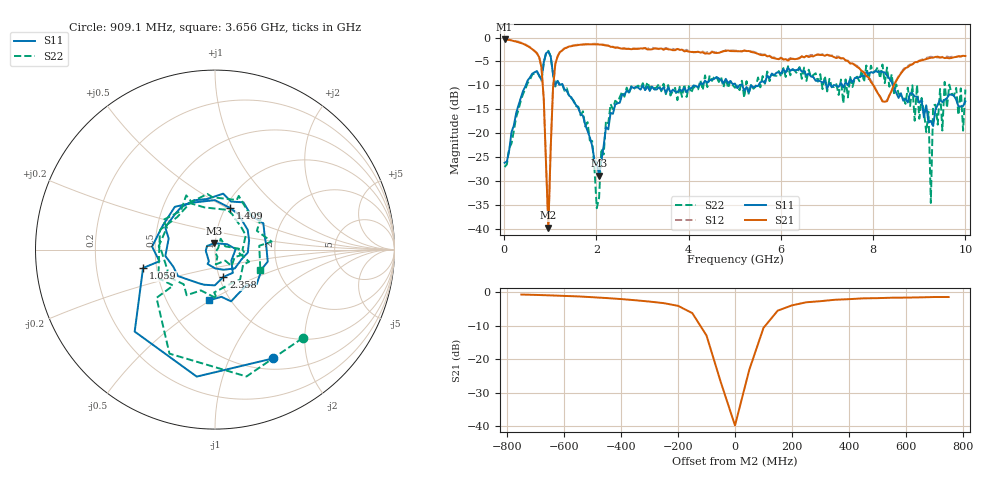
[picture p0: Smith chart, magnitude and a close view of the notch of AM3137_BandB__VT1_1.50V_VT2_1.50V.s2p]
! Date/Time: Tue, Nov 13, 2018 4:51 PM
! Network Analyzer: Agilent Technologies E8364B Rev: A.07.50.67
! Sweep from 0.010 to 10.000 GHz, 201 Points, Sweep Type: LIN
! Power Supply: 1.501 V, 0.000 A
# Hz S DB R 50
!freq MagS11 AngS11 MagS21 AngS21 MagS12 AngS12 MagS22 AngS22
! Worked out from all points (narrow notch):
!   201 points, 10 MHz to 10 GHz, reference 50 ohm
!   highest |S21| = -0.35 dB at 10 MHz (marker M1); lowest = -39.8 dB at 959 MHz (marker M2)
!   notch at M2: 36.4 dB deep, 125 MHz wide at half that depth
!   lowest |S11| = -28.9 dB at 2.058 GHz (marker M3), VSWR 1.07, Z = 49.5 + j3.52 ohm
!   |S11| at or under -10 dB: start of sweep to 468.6 MHz; 1.272 GHz to 4.23 GHz (2.958 GHz wide, 108 % of centre); 8.429 GHz to end of sweep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
!   |S22| runs from -35.7 to -2.8 dB; largest |S21 - S12| = 0.034
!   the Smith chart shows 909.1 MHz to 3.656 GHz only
!   S11 on the Smith chart (normalised r, x): 909.1 MHz: 0.64, -1.47; 1.059 GHz: 0.42, -0.10; 1.409 GHz: 1.05, +0.52; 2.358 GHz: 1.05, -0.33; 3.656 GHz: 0.80, -0.49
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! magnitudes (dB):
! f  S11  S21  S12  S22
! 10 MHz  -26.2  -0.4  -0.3  -27.1
! 759.2 MHz  -7.9  -4.1  -4.0  -8.0
! 909.1 MHz  -3.3  -26.8  -26.6  -3.2
! 959 MHz  -2.9  -39.8  -39.8  -2.8
! 1.059 GHz  -7.7  -10.7  -10.6  -7.5
! 1.409 GHz  -12.2  -1.9  -1.8  -12.3
! 1.708 GHz  -16.3  -1.5  -1.4  -15.4
! 2.058 GHz  -28.9  -1.4  -1.3  -33.6
! 2.108 GHz  -25.8  -1.5  -1.4  -23.2
! 2.358 GHz  -16.0  -2.0  -1.9  -15.0
! 3.357 GHz  -10.4  -2.3  -2.4  -9.7
! 3.656 GHz  -10.9  -2.6  -2.4  -11.1
! 5.005 GHz  -9.6  -2.8  -2.7  -10.5
! 6.703 GHz  -8.3  -3.9  -3.6  -7.8
! 8.352 GHz  -8.5  -12.1  -12.1  -10.3
! 9.201 GHz  -17.8  -4.3  -4.1  -15.5
! 9.251 GHz  -17.4  -4.2  -4.0  -34.6
! 9.301 GHz  -18.5  -4.2  -4.1  -14.2
! 9.5 GHz  -13.5  -4.1  -4.0  -19.5
! 9.9 GHz  -14.4  -3.9  -4.0  -10.6
! 9.95 GHz  -14.4  -3.8  -3.8  -19.5
! 10 GHz  -13.4  -3.9  -3.8  -10.9
